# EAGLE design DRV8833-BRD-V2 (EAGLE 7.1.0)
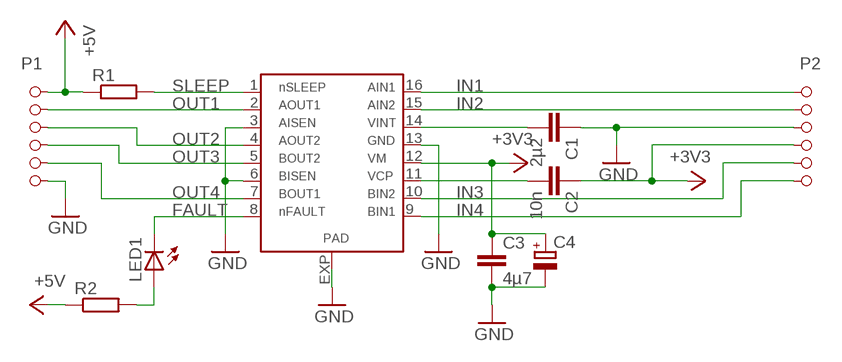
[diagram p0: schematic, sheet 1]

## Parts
C1  2µ2  C-EUC1206  [C1206]
C2  10n  C-EUC1206  [C1206]
C3  4µ7  C-EUC1206  [C1206]
C4  CPOL-EU153CLV-0605  [153CLV-0605]
IC1  DRV8833  [HTSSOP16PWP]
LED1  LEDSMT1206  [1206]
P1  SMD-6  [SMD-6]
P2  SMD-6  [SMD-6]
R1  R-EU_R1206  [R1206]
R2  R-EU_R1206  [R1206]

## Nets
+3V3: C2.1 C3.1 C4.+ IC1.12 P2.P$4
+5V: P1.P$1 R1.1 R2.1
FAULT: IC1.8 LED1.C
GND: C1.1 C3.2 C4.- IC1.3 IC1.6 IC1.13 IC1.EXP P1.P$6 P2.P$3
IN1: IC1.16 P2.P$1
IN2: IC1.15 P2.P$2
IN3: IC1.10 P2.P$5
IN4: IC1.9 P2.P$6
N$1: C1.2 IC1.14
N$3: C2.2 IC1.11
N$5: LED1.A R2.2
OUT1: IC1.2 P1.P$2
OUT2: IC1.4 P1.P$3
OUT3: IC1.5 P1.P$4
OUT4: IC1.7 P1.P$5
SLEEP: IC1.1 R1.2

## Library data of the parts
C1-C3 = rcl:C-EU: CAPACITOR, European symbol
C4 = rcl:CPOL-EU: POLARIZED CAPACITOR, European symbol
IC1 = 1Axel:DRV8833
LED1 = led:LED: LED
P1 P2 = PinHeader:SMD-6
R1 R2 = rcl:R-EU_: RESISTOR, European symbol

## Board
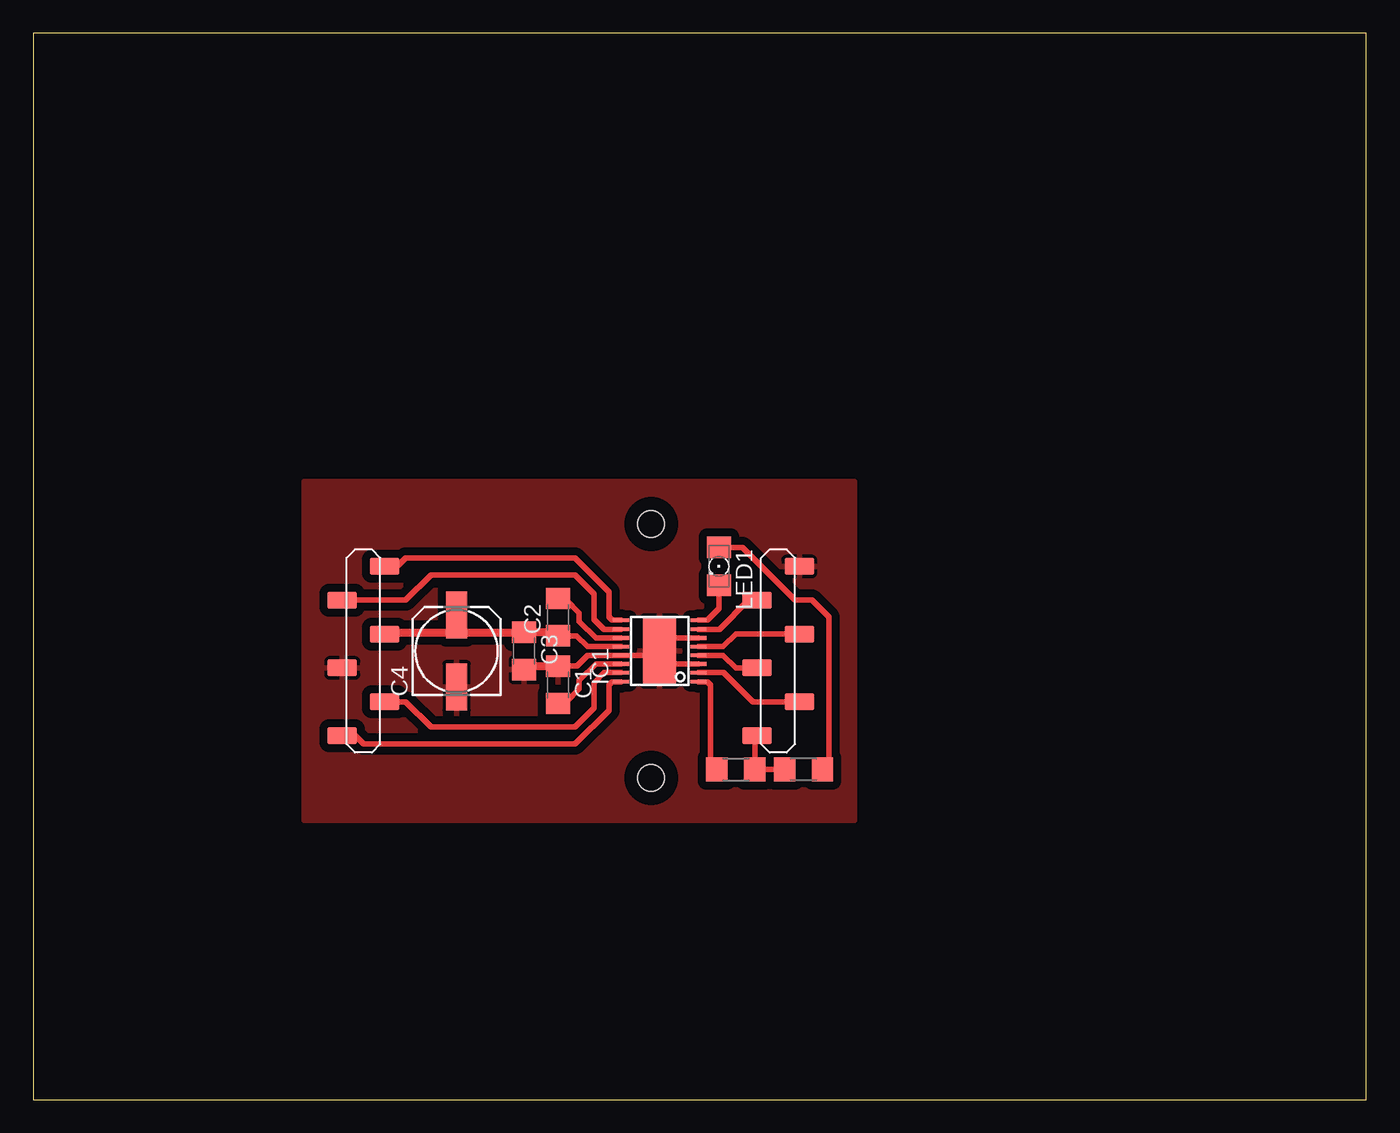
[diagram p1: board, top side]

Size 100 x 80 mm. Coordinates in mm from the lower left corner, seen from the top.
Outline: 0,0 100,0 100,80 0,80 0,0
Copper layers (1*16): Top 0.035mm / dielectric 1.5mm / Bottom 0.035mm
Design rules "default": minimum track width 10mil, minimum drill 24mil, track to track 8mil, track to pad 8mil, pad to pad 8mil, via to via 8mil, smd to smd 8mil, copper to edge 40mil, drill to drill 8mil, minimum pad ring 10mil, minimum via ring 8mil, stop-mask expansion 4mil, vias tented up to drill 0mil, thermal gap 10mil
Holes 2 mm at 46.35,43.18 46.35,24.13
tRestrict: area 36.8,32.4 to 41.3,35.6

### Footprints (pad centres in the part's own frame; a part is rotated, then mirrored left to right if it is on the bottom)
C1206 = smd 1.6 x 1.8: 1 -1.4,0; 2 1.4,0
153CLV-0605 = smd 3.5 x 1.6: + 2.7,0; - -2.7,0
HTSSOP16PWP = smd 0.27 x 1.2: 1 -3.588,-2.9; 2 -2.895,-2.9; 3 -2.245,-2.9; 4 -1.595,-2.9; 5 -0.945,-2.9; 6 -0.295,-2.9; 7 0.355,-2.9; 8 1.048,-2.9; 9 1.048,2.9; 10 0.355,2.9; 11 -0.295,2.9; 12 -0.945,2.9; 13 -1.595,2.9; 14 -2.245,2.9; 15 -2.895,2.9; 16 -3.588,2.9 | smd 5.08 x 2.46: EXP -1.27,0
1206 = smd 1.6 x 1.803: A -1.422,0; C 1.422,0
SMD-6 = smd 1.27 x 2.2: P$1 -6.35,1.587; P$2 -3.81,-1.587; P$3 -1.27,1.587; P$4 1.27,-1.587; P$5 3.81,1.587; P$6 6.35,-1.587
R1206 = smd 1.6 x 1.803: 1 -1.422,0; 2 1.422,0

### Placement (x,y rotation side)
C1  39.37,31.11 270 top
C2  39.37,36.2 90 top
C3  36.83,33.66 270 top
C4  31.75,33.66 90 top
IC1  46.99,34.92 90 top
LED1  51.44,40.01 270 top
P1  55.88,33.66 90 top
P2  24.77,33.66 90 top
R1  52.7,24.77 180 top
R2  57.78,24.77 0 top

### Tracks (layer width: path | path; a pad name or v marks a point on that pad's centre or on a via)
+3V3
  Top 0.406: IC1.12 41.59,33.98 40.77,34.8 C2.1 39.37,35.05 | P2.P$4 26.35,35.05 | C4.+ 31.75,35.05
  Top 0.61: 39.37,35.05 C3.1 31.75,35.05 26.35,35.05
+5V
  Top 0.406: P1.P$1 54.13,27.14 R1.1 R2.1
FAULT
  Top 0.406: IC1.8 50.58,35.97 51.44,36.83 LED1.C
GND
  Top 0.305: 46.99,32.68 IC1.EXP | 46.99,34.63 IC1.EXP | 46.99,33.33 IC1.EXP | 39.34,32.54 C1.1
  Top 0.406: 39.34,32.54 40.8,32.54 41.59,33.33 IC1.13 46.99,33.33 | IC1.3 46.99,32.68 | IC1.6 46.99,34.63
  Top 0.61: C3.2 37.09,32.52 C1.1
  pour Top (isolate 0.61): 20.32,20.95 20.32,46.35 61.59,46.35 61.59,20.95
IN1
  Top 0.406: IC1.16 43.4,31.34 43.18,31.11 43.18,29.21 40.64,26.67 24.77,26.67 24.13,27.3 P2.P$1
IN2
  Top 0.406: IC1.15 42.83,32.03 42.07,31.27 42.07,29.37 40.64,27.94 29.84,27.94 27.94,29.84 P2.P$2
IN3
  Top 0.406: IC1.10 42.83,35.28 42.07,36.04 42.07,37.94 40.64,39.37 29.84,39.37 27.94,37.47 P2.P$5
IN4
  Top 0.406: IC1.9 43.4,35.97 43.18,36.2 43.18,38.1 40.64,40.64 27.94,40.64 27.3,40.01 P2.P$6
N$1
  Top 0.305: 40.01,29.84 39.5,29.84 C1.2
  Top 0.406: IC1.14 42.2,32.68 40.96,31.43 40.96,30.8 40.01,29.84
N$2  (via drill 0.6)
  other vias: 46.35,43.18
N$3
  Top 0.305: 40.01,37.47 39.5,37.47 C2.2
  Top 0.406: IC1.11 42.2,34.63 40.96,35.88 40.96,36.51 40.01,37.47
N$4  (via drill 0.6)
  other vias: 46.35,24.13
N$5
  Top 0.406: LED1.A 53.19,41.43 57.15,37.47 58.42,37.47 59.69,36.2 59.69,25.25 R2.2
OUT1
  Top 0.406: P1.P$2 53.98,29.84 51.79,32.03 IC1.2
OUT2
  Top 0.406: IC1.4 51.76,33.33 52.7,32.38 P1.P$3
OUT3
  Top 0.406: IC1.5 51.76,33.98 52.7,34.92 P1.P$4
OUT4
  Top 0.305: P1.P$5 53.66,37.47
  Top 0.406: IC1.7 51.47,35.28 53.66,37.47
SLEEP
  Top 0.406: IC1.1 50.58,31.34 50.8,31.11 50.8,25.25 R1.2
